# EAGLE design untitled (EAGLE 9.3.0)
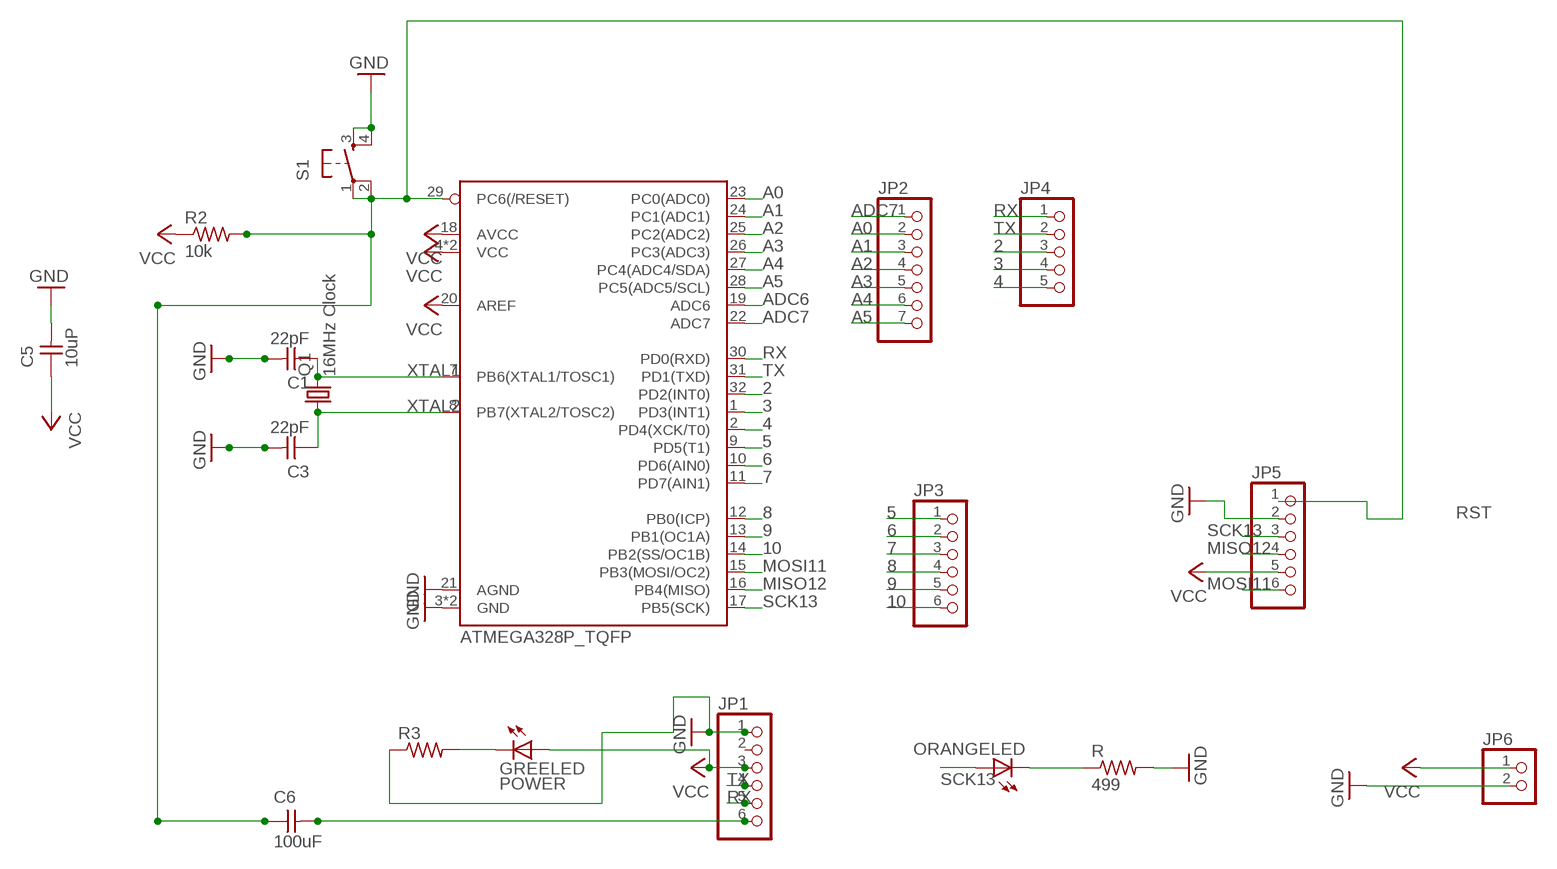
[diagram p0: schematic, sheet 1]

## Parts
C1  22pF  CAP-UNPOLARIZEDFAB  [C1206FAB]
C3  22pF  CAP-UNPOLARIZEDFAB  [C1206FAB]
C5  10uP  CAP-UNPOLARIZEDFAB  [C1206FAB]
C6  100uF  CAP-UNPOLARIZEDFAB  [C1206FAB]
GREELED  POWER  LEDFAB1206  [LED1206FAB]
JP1  PINHD-1X6  [1X06]
JP2  PINHD-1X7  [1X07]
JP3  PINHD-1X6  [1X06]
JP4  PINHD-1X5  [1X05]
JP5  PINHD-1X6  [1X06]
JP6  PINHD-1X2  [1X02]
ORANGELED  SCK  LEDFAB1206  [LED1206FAB]
Q1  16MHz Clock  CSM-7X-DU  [CSM-7X-DU]
R  499  RES-US1206FAB  [R1206FAB]
R2  10k  RES-US1206FAB  [R1206FAB]
R3  RES-US1206FAB  [R1206FAB]
S1  6MM_SWITCH6MM_SWITCH  [6MM_SWITCH]
U2  ATMEGA328P_TQFP  [TQFP32-08]

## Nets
2: JP4.3 U2.32(PD2(INT0))
3: JP4.4 U2.1(PD3(INT1))
4: JP4.5 U2.2(PD4(XCK/T0))
5: JP3.1 U2.9(PD5(T1))
6: JP3.2 U2.10(PD6(AIN0))
7: JP3.3 U2.11(PD7(AIN1))
8: JP3.4 U2.12(PB0(ICP))
9: JP3.5 U2.13(PB1(OC1A))
10: JP3.6 U2.14(PB2(SS/OC1B))
A0: JP2.2 U2.23(PC0(ADC0))
A1: JP2.3 U2.24(PC1(ADC1))
A2: JP2.4 U2.25(PC2(ADC2))
A3: JP2.5 U2.26(PC3(ADC3))
A4: JP2.6 U2.27(PC4(ADC4/SDA))
A5: JP2.7 U2.28(PC5(ADC5/SCL))
ADC6: U2.19(ADC6)
ADC7: JP2.1 U2.22(ADC7)
GND: C1.2 C3.2 C5.2 JP1.1 JP5.2 JP6.2 R3.1 R.2 S1.3(S) S1.4(S1) U2.3(GND) U2.5(GND) U2.21(AGND)
MISO12: JP5.4 U2.16(PB4(MISO))
MOSI11: JP5.6 U2.15(PB3(MOSI/OC2))
N$1: C6.2 JP1.6
N$26: ORANGELED.2(C) R.1
N$28: GREELED.2(C) R3.2
RST: C6.1 JP5.1 R2.2 S1.1(P) S1.2(P1) U2.29(PC6(/RESET))
RX: JP1.5 JP4.1 U2.30(PD0(RXD))
SCK13: JP5.3 ORANGELED.1(A) U2.17(PB5(SCK))
TX: JP1.4 JP4.2 U2.31(PD1(TXD))
VCC: C5.1 GREELED.1(A) JP1.3 JP5.5 JP6.1 R2.1 U2.4(VCC) U2.6(VCC) U2.18(AVCC) U2.20(AREF)
XTAL1: C1.1 Q1.2 U2.7(PB6(XTAL1/TOSC1))
XTAL2: C3.1 Q1.1 U2.8(PB7(XTAL2/TOSC2))
Unconnected: JP1.2

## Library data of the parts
C1 C3 C5 C6 = fab:CAP-UNPOLARIZED
GREELED ORANGELED = fab:LED: LED
JP1 JP3 JP5 = pinhead:PINHD-1X6: PIN HEADER
JP2 = pinhead:PINHD-1X7: PIN HEADER
JP4 = pinhead:PINHD-1X5: PIN HEADER
JP6 = pinhead:PINHD-1X2: PIN HEADER
Q1 = crystal:CSM-7X-DU: SMD CRYSTAL; OC_FARNELL: unknown; OC_NEWARK: unknown
R R2 R3 = fab:RES-US: Resistor (US Symbol)
S1 = fab:6MM_SWITCH: OMRON SWITCH
U2 = SparkFun-IC-Microcontroller:ATMEGA328P_TQFP: Popular 328P in QFP Storefront component: ATmega328 - TQFP (COM-13448) Datasheet SparkFun Products SparkFun RedBoard - Programmed with Arduino (DEV-12757) Arduino Pro Mini 328 - 5V/16MHz (DEV-11113) Arduino Pro Mini 328 - 3.3V/8MHz (DEV-11114) SparkFun OpenLog (DEV-13712) SparkFun MicroView - OLED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; PROD_ID: IC-09069

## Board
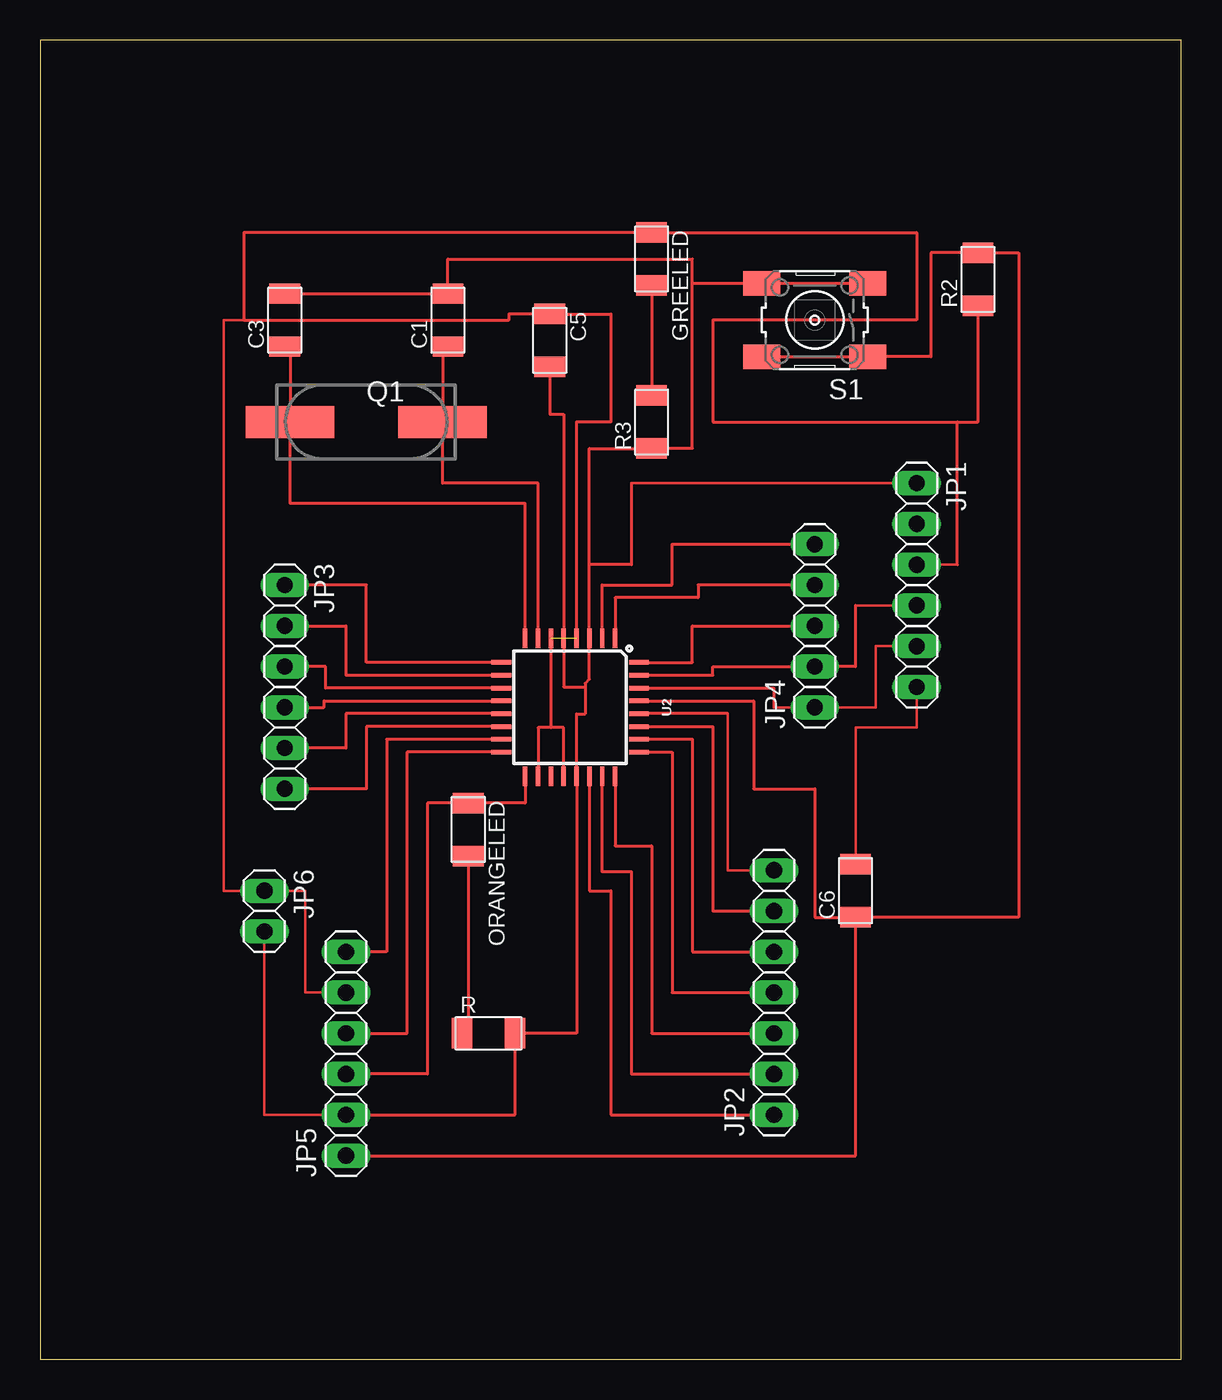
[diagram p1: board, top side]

Size 71.1 x 82.22 mm. Coordinates in mm from the lower left corner, seen from the top.
Outline: 0,0 71.1,0 71.1,82.22 0,82.22 0,0
Copper layers (1*16): Top 0.035mm / dielectric 1.5mm / Bottom 0.035mm
Design rules "default": minimum track width 6mil, minimum drill 0.35mm, track to track 6mil, track to pad 6mil, pad to pad 6mil, via to via 6mil, smd to smd 6mil, copper to edge 40mil, drill to drill 6mil, minimum pad ring 10mil, minimum via ring 8mil, stop-mask expansion 4mil, vias tented up to drill 0mil, thermal gap 10mil

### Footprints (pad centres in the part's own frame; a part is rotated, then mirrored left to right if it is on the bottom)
C1206FAB = smd 1.27 x 1.905: 1 -1.651,0; 2 1.651,0
LED1206FAB = smd 1.27 x 1.905: 1 -1.651,0; 2 1.651,0
1X06 = drill 1.016 long: 1 -6.35,0; 2 -3.81,0; 3 -1.27,0; 4 1.27,0; 5 3.81,0; 6 6.35,0
1X07 = drill 1.016 long: 1 -7.62,0; 2 -5.08,0; 3 -2.54,0; 4 0,0; 5 2.54,0; 6 5.08,0; 7 7.62,0
1X05 = drill 1.016 long: 1 -5.08,0; 2 -2.54,0; 3 0,0; 4 2.54,0; 5 5.08,0
1X02 = drill 1.016 long: 1 -1.27,0; 2 1.27,0
CSM-7X-DU = smd 5.5 x 2: 1 -4.75,0; 2 4.75,0
R1206FAB = smd 1.27 x 1.905: 1 -1.651,0; 2 1.651,0
6MM_SWITCH = smd 2.286 x 1.524: 1 -3.302,2.286; 2 3.302,2.286; 3 -3.302,-2.286; 4 3.302,-2.286
TQFP32-08 = smd 1.219 x 0.279: 1 -4.293,2.8; 2 -4.293,2; 3 -4.293,1.2; 4 -4.293,0.4; 5 -4.293,-0.4; 6 -4.293,-1.2; 7 -4.293,-2; 8 -4.293,-2.8; 17 4.293,-2.8; 18 4.293,-2; 19 4.293,-1.2; 20 4.293,-0.4; 21 4.293,0.4; 22 4.293,1.2; 23 4.293,2; 24 4.293,2.8 | smd 0.279 x 1.219: 9 -2.8,-4.293; 10 -2,-4.293; 11 -1.2,-4.293; 12 -0.4,-4.293; 13 0.4,-4.293; 14 1.2,-4.293; 15 2,-4.293; 16 2.8,-4.293; 25 2.8,4.293; 26 2,4.293; 27 1.2,4.293; 28 0.4,4.293; 29 -0.4,4.293; 30 -1.2,4.293; 31 -2,4.293; 32 -2.8,4.293

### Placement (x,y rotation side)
C1  25.4,64.77 90 top
C3  15.24,64.77 90 top
C5  31.75,63.5 270 top
C6  50.8,29.21 90 top
GREELED  38.1,68.58 270 top
JP1  54.61,48.26 270 top
JP2  45.72,22.86 90 top
JP3  15.24,41.91 270 top
JP4  48.26,45.72 90 top
JP5  19.05,19.05 90 top
JP6  13.97,27.94 270 top
ORANGELED  26.67,33.02 270 top
Q1  20.32,58.42 0 top
R  27.94,20.32 0 top
R2  58.42,67.31 90 top
R3  38.1,58.42 90 top
S1  48.26,64.77 180 top
U2  33.02,40.64 270 top

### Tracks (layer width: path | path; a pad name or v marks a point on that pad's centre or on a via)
2
  Top 0.2: JP4.3 40.64,45.72 40.64,43.44 U2.32
3
  Top 0.2: JP4.4 40.99,48.26 40.99,47.47 35.82,47.47 U2.1
4
  Top 0.2: U2.2 35.02,48.26 39.37,48.26 39.37,50.8 JP4.5
5
  Top 0.2: JP3.1 20.32,48.26 20.32,43.44 U2.9
6
  Top 0.2: JP3.2 19.05,45.72 19.05,42.64 U2.10
7
  Top 0.2: JP3.3 17.78,43.18 17.78,41.84 U2.11
8
  Top 0.2: JP3.4 17.68,40.64 17.68,41.04 U2.12
9
  Top 0.2: U2.13 19.05,40.24 19.05,38.1 JP3.5
10
  Top 0.2: JP3.6 20.32,35.56 20.32,39.44 U2.14
A0
  Top 0.2: U2.23 35.02,30.38 36.83,30.38 36.83,17.78 JP2.2
A1
  Top 0.2: U2.24 35.82,32 38.1,32 38.1,20.32 JP2.3
A2
  Top 0.2: U2.25 39.37,37.84 39.37,22.86 JP2.4
A3
  Top 0.2: U2.26 40.64,38.64 40.64,25.4 JP2.5
A4
  Top 0.2: JP2.6 41.91,27.94 41.91,39.44 U2.27
A5
  Top 0.152: JP2.7 42.83,30.48 42.83,40.24
  Top 0.2: 42.83,40.24 U2.28
ADC7
  Top 0.2: JP2.1 35.56,15.24 35.56,29.21 34.22,29.21 U2.22
GND
  Top 0.152: JP1.1 36.83,54.61 | JP6.2 13.97,15.24 JP5.2
  Top 0.2: 36.83,54.61 36.83,49.53 34.22,49.53 | C5.2 31.75,58.9 32.62,58.9 U2.5 32.62,41.91 33.95,41.91 | C3.2 C1.2 25.4,68.58 40.64,68.58 40.64,67.06 | S1.3 S1.4 40.64,67.06 | 33.95,41.91 33.95,42.12 34.22,42.39 U2.3 34.22,49.53 | 33.95,41.91 33.95,40.23 33.42,40.23 U2.21 33.42,20.32 R.2 29.59,15.24 JP5.2 | 40.64,67.06 40.64,56.77 R3.1 34.22,56.77 34.22,49.53
MISO12
  Top 0.2: JP5.4 22.86,20.32 22.86,37.84 U2.16
MOSI11
  Top 0.2: U2.15 21.59,38.64 21.59,25.4 JP5.6
N$1
  Top 0.152: JP1.6 54.61,39.37 50.8,39.37 C6.2
N$26
  Top 0.2: ORANGELED.2 26.67,20.32 R.1
N$28
  Top 0.2: GREELED.2 R3.2
RST
  Top 0.2: U2.29 44.45,41.04 44.45,35.56 48.26,35.56 48.26,27.56 C6.1 | S1.2 S1.1 55.5,62.48 55.5,68.96 R2.2 60.96,68.96 60.96,27.56 C6.1 | JP5.1 50.8,12.7 C6.1
RX
  Top 0.152: JP1.5 52.07,44.45 52.07,40.64 JP4.1 45.72,40.64 | U2.30 37.31,41.91
  Top 0.2: U2.30 45.72,41.84 45.72,40.64
SCK13
  Top 0.2: JP5.3 24.13,17.78 24.13,34.67 ORANGELED.1 30.22,34.67 U2.17
TX
  Top 0.152: 50.8,46.99 JP1.4
  Top 0.2: U2.31 41.91,42.64 41.91,43.18 JP4.2 50.8,43.18 50.8,46.99
VCC  (1 unrouted)
  Top 0.152: JP1.3 57.15,49.53 | JP5.5 16.51,22.86 16.51,29.21 JP6.1 11.43,29.21 11.43,64.77 12.7,64.77
  Top 0.2: U2.6 31.82,39.37 | 31.82,39.37 31.02,39.37 U2.18 | U2.4 33.42,58.42 35.56,58.42 35.56,65.15 C5.1 29.21,65.15 29.21,64.77 12.7,64.77 12.7,70.23 GREELED.1 54.61,70.23 54.61,64.77 41.91,64.77 41.91,58.42 57.15,58.42 | 57.15,49.53 57.15,58.42 | R2.1 58.42,58.42 57.15,58.42 | U2.20 32.62,39.37 31.82,39.37
XTAL1
  Top 0.2: U2.7 31.02,54.61 25.07,54.61 Q1.2 25.07,63.12 C1.1
XTAL2
  Top 0.2: U2.8 30.22,53.34 15.57,53.34 Q1.1 15.57,63.12 C3.1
